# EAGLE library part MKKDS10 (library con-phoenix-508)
PHOENIX
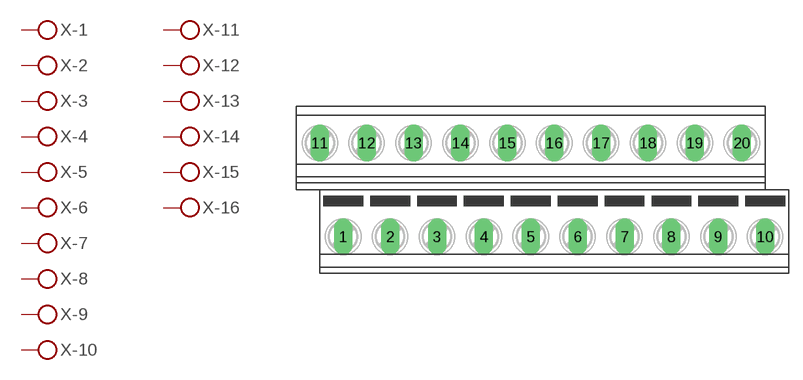
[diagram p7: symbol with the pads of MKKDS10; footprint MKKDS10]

Designator prefix X; gates -1=KL -2=KL -3=KL -4=KL -5=KL -6=KL -7=KL -8=KL -9=KL -10=KL -11=KL -12=KL -13=KL -14=KL -15=KL -16=KL -17=KL -18=KL -19=KL -20=KLV

## MKKDS10 (OC_FARNELL: unknown; OC_NEWARK: unknown)  [MKKDS10]
1  -1:KL  pas
2  -2:KL  pas
3  -3:KL  pas
4  -4:KL  pas
5  -5:KL  pas
6  -6:KL  pas
7  -7:KL  pas
8  -8:KL  pas
9  -9:KL  pas
10  -10:KL  pas
11  -11:KL  pas
12  -12:KL  pas
13  -13:KL  pas
14  -14:KL  pas
15  -15:KL  pas
16  -16:KL  pas
17  -17:KL  pas
18  -18:KL  pas
19  -19:KL  pas
20  -20:KL  pas

## Footprint MKKDS10 (pad centres in mm)
PHOENIX MKKDSN 1,5/ 8-5,08 Source: http://eshop.phoenixcontact.com .. 1726202.pdf
drill 1.321 long: 1 -21.59,-5.08; 2 -16.51,-5.08; 3 -11.43,-5.08; 4 -6.35,-5.08; 5 -1.27,-5.08; 6 3.81,-5.08; 7 8.89,-5.08; 8 13.97,-5.08; 9 19.05,-5.08; 10 24.13,-5.08; 11 -24.13,5.08; 12 -19.05,5.08; 13 -13.97,5.08; 14 -8.89,5.08; 15 -3.81,5.08; 16 1.27,5.08; 17 6.35,5.08; 18 11.43,5.08; 19 16.51,5.08; 20 21.59,5.08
